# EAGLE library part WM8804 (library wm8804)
TRANSCEIVER, S/PDIF, 1:1, 20SSOP Supply Voltage Range: 2.7V to 3.6V Logic Case Style: SSOP No. of Pins: 20 Operating Temperature Range: -40°C to +85°C SVHC: No SVHC (19-Dec-2011) Interface Type: Serial, 2 / 3 Wire Line / Bus Driver / Receiver / Transceiver Type: Digital Interface Transceiver with PLL No. of Channels: 2 Package / Case: SSOP Supply Current: 14.9mA Supply Voltage Max: 3.6V Supply Voltage Min: 2.7V Termination Type: SMD datasheet
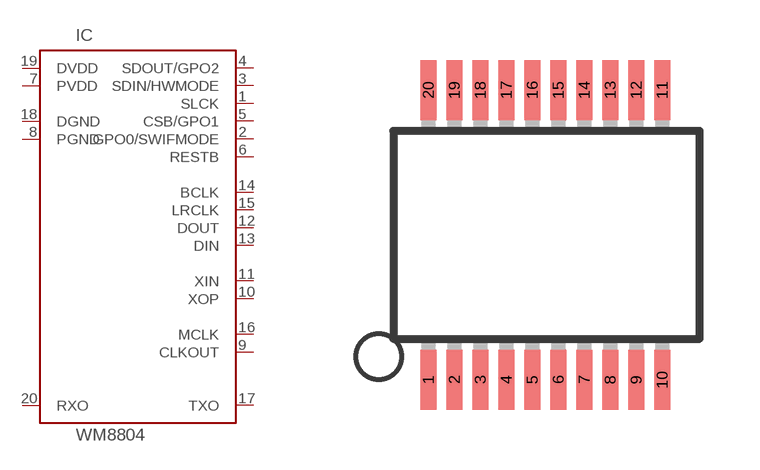
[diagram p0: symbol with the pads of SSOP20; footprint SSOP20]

Designator prefix IC

## WM8804  [SSOP20]
1  SLCK  in
2  GPO0/SWIFMODE  out
3  SDIN/HWMODE  in
4  SDOUT/GPO2  out
5  CSB/GPO1  in
6  RESTB  in
7  PVDD  pwr
8  PGND  pwr
9  CLKOUT  out
10  XOP
11  XIN
12  DOUT  out
13  DIN  in
14  BCLK
15  LRCLK
16  MCLK
17  TXO  out
18  DGND  pwr
19  DVDD  pwr
20  RXO  in

## Footprint SSOP20 (pad centres in mm)
smd 0.4 x 1.5: 1 -2.955,-3.625; 2 -2.305,-3.625; 3 -1.655,-3.625; 4 -1.005,-3.625; 5 -0.355,-3.625; 6 0.295,-3.625; 7 0.945,-3.625; 8 1.595,-3.625; 9 2.245,-3.625; 10 2.895,-3.625; 11 2.895,3.625; 12 2.245,3.625; 13 1.595,3.625; 14 0.945,3.625; 15 0.295,3.625; 16 -0.355,3.625; 17 -1.005,3.625; 18 -1.655,3.625; 19 -2.305,3.625; 20 -2.955,3.625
